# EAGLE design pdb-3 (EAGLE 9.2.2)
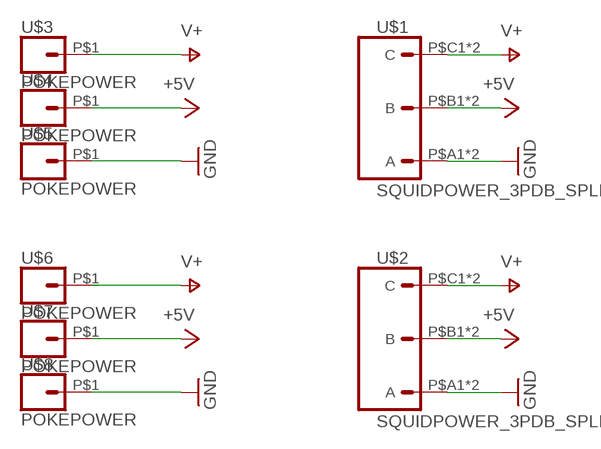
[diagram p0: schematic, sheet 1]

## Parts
U$1  SQUIDPOWER_3PDB_SPLIT  [PDBCONN_ABC]
U$2  SQUIDPOWER_3PDB_SPLIT  [PDBCONN_ABC]
U$3  POKEPOWER  [LITE-TRAP-MOLEX-203863]
U$4  POKEPOWER  [LITE-TRAP-MOLEX-203863]
U$5  POKEPOWER  [LITE-TRAP-MOLEX-203863]
U$6  POKEPOWER  [LITE-TRAP-MOLEX-203863]
U$7  POKEPOWER  [LITE-TRAP-MOLEX-203863]
U$8  POKEPOWER  [LITE-TRAP-MOLEX-203863]

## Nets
+5V: U$1.P$B1(B) U$1.P$B2(B) U$2.P$B1(B) U$2.P$B2(B) U$4.P$1 U$7.P$1
GND: U$1.P$A1(A) U$1.P$A2(A) U$2.P$A1(A) U$2.P$A2(A) U$5.P$1 U$8.P$1
V+: U$1.P$C1(C) U$1.P$C2(C) U$2.P$C1(C) U$2.P$C2(C) U$3.P$1 U$6.P$1

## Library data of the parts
U$1 U$2 = connector:SQUIDPOWER_3
U$3-U$8 = connector:POKEPOWER

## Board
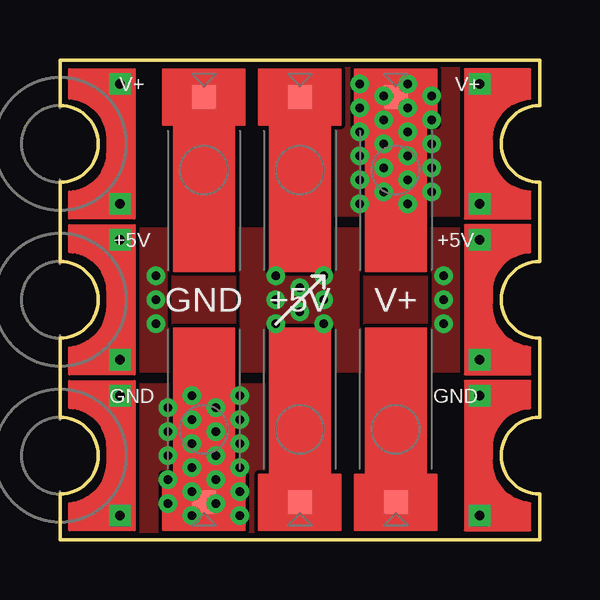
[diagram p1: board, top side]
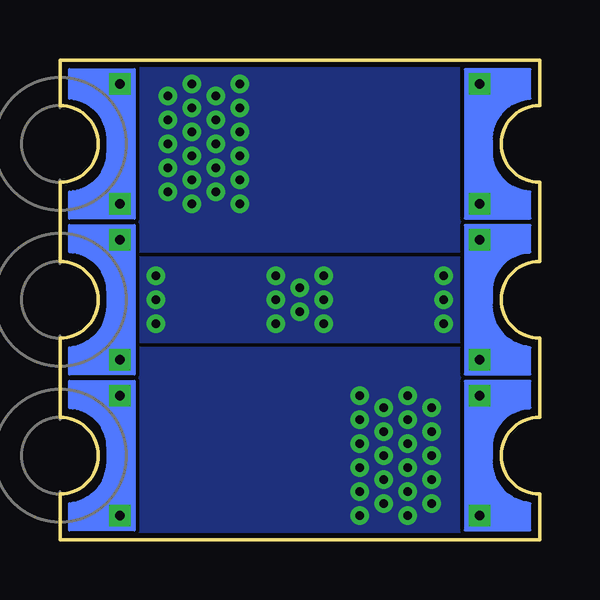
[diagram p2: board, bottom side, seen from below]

Size 20 x 20 mm. Coordinates in mm from the lower left corner, seen from the top.
Outline: 0,5.1 0,8.4 arc90 1.6,10 arc90 0,11.6 0,14.9 arc90 1.6,16.5 arc90 0,18.1 0,20 20,20 20,18.1 arc90 18.4,16.5 arc90 20,14.9 20,11.6 arc90 18.4,10 arc90 20,8.4 20,5.1 arc90 18.4,3.5 arc90 20,1.9 20,0 0,0 0,1.9 arc90 1.6,3.5 arc90 0,5.1
Copper layers (1*16): Top 0.035mm / dielectric 1.5mm / Bottom 0.035mm
Design rules "default *": minimum track width 6mil, minimum drill 0.35mm, track to track 6mil, track to pad 6mil, pad to pad 6mil, via to via 6mil, smd to smd 6mil, copper to edge 8mil, drill to drill 6mil, minimum pad ring 10mil, minimum via ring 8mil, stop-mask expansion 4mil, vias tented up to drill 0mil, thermal gap 10mil

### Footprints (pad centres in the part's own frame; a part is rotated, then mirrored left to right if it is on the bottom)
PDBCONN_ABC = drill 0.4 square: P$A1 2.5,-9; P$A2 2.5,-4; P$B1 2.5,-2.5; P$B2 2.5,2.5; P$C1 2.5,4; P$C2 2.5,9
LITE-TRAP-MOLEX-203863 = smd 1 x 1: P$1 -3.05,0

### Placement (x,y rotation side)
U$1  20,10 0 bottom
U$2  0,10 0 top
U$3  14,4.6 90 top
U$4  10,4.6 90 top
U$5  6,4.6 90 top
U$6  14,15.4 270 top
U$7  10,15.4 270 top
U$8  6,15.4 270 top

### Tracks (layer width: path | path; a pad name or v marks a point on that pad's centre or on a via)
+5V  (via drill 0.35)
  other vias: 10,9.5 10,10.5 11,10 11,11 11,9 9,9 9,10 9,11 4,10 16,10 16,11 16,9 4,9 4,11
  pour Top (rank 5, no thermals): 9,18.5 9,12 8.5,11.5 8.5,8.5 9,8 9,1.5 11,1.5 11,8 11.5,8.5 11.5,11.5 11,12 11,18.5
  pour Bottom (rank 6, no thermals): -3.5,12 23.5,12 23.5,8 -3.5,8
  pour Top (rank 6, no thermals): -1,13 21,13 21,7 -1,7
GND  (via drill 0.35)
  other vias: 7.5,6 7.5,5 7.5,4 7.5,3 6.5,3.5 6.5,4.5 6.5,5.5 5.5,6 5.5,5 5.5,4 5.5,3 6.5,2.5 7.5,2 7.5,1 6.5,1.5 5.5,2 5.5,1 4.5,5.5 4.5,4.5 4.5,3.5 4.5,2.5 4.5,1.5
  pour Bottom (rank 2, no thermals): -3.5,8 23.5,8 23.5,-1 -3.5,-1
  pour Top (rank 6, no thermals): -1,6.5 21,6.5 21,-0.5 -1,-0.5
  pour Top (rank 5, no thermals): 7.3,18.5 7.3,1.5 4.7,1.5 4.7,18.5
V+  (via drill 0.35)
  other vias: 12.5,14 12.5,15 12.5,16 12.5,17 13.5,16.5 13.5,15.5 13.5,14.5 14.5,14 14.5,15 14.5,16 14.5,17 13.5,17.5 12.5,18 12.5,19 13.5,18.5 14.5,18 14.5,19 15.5,14.5 15.5,15.5 15.5,16.5 15.5,17.5 15.5,18.5
  pour Bottom (rank 2, no thermals): -3.5,12 23.5,12 23.5,21 -3.5,21
  pour Top (rank 6, no thermals): -1,21 21,21 21,13.5 -1,13.5
  pour Top (rank 5, no thermals): 12.7,1.5 12.7,18.5 15.3,18.5 15.3,1.5

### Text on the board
tPlace: V+ | V+ | +5V | +5V | GND | +5V | V+ | GND | GND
